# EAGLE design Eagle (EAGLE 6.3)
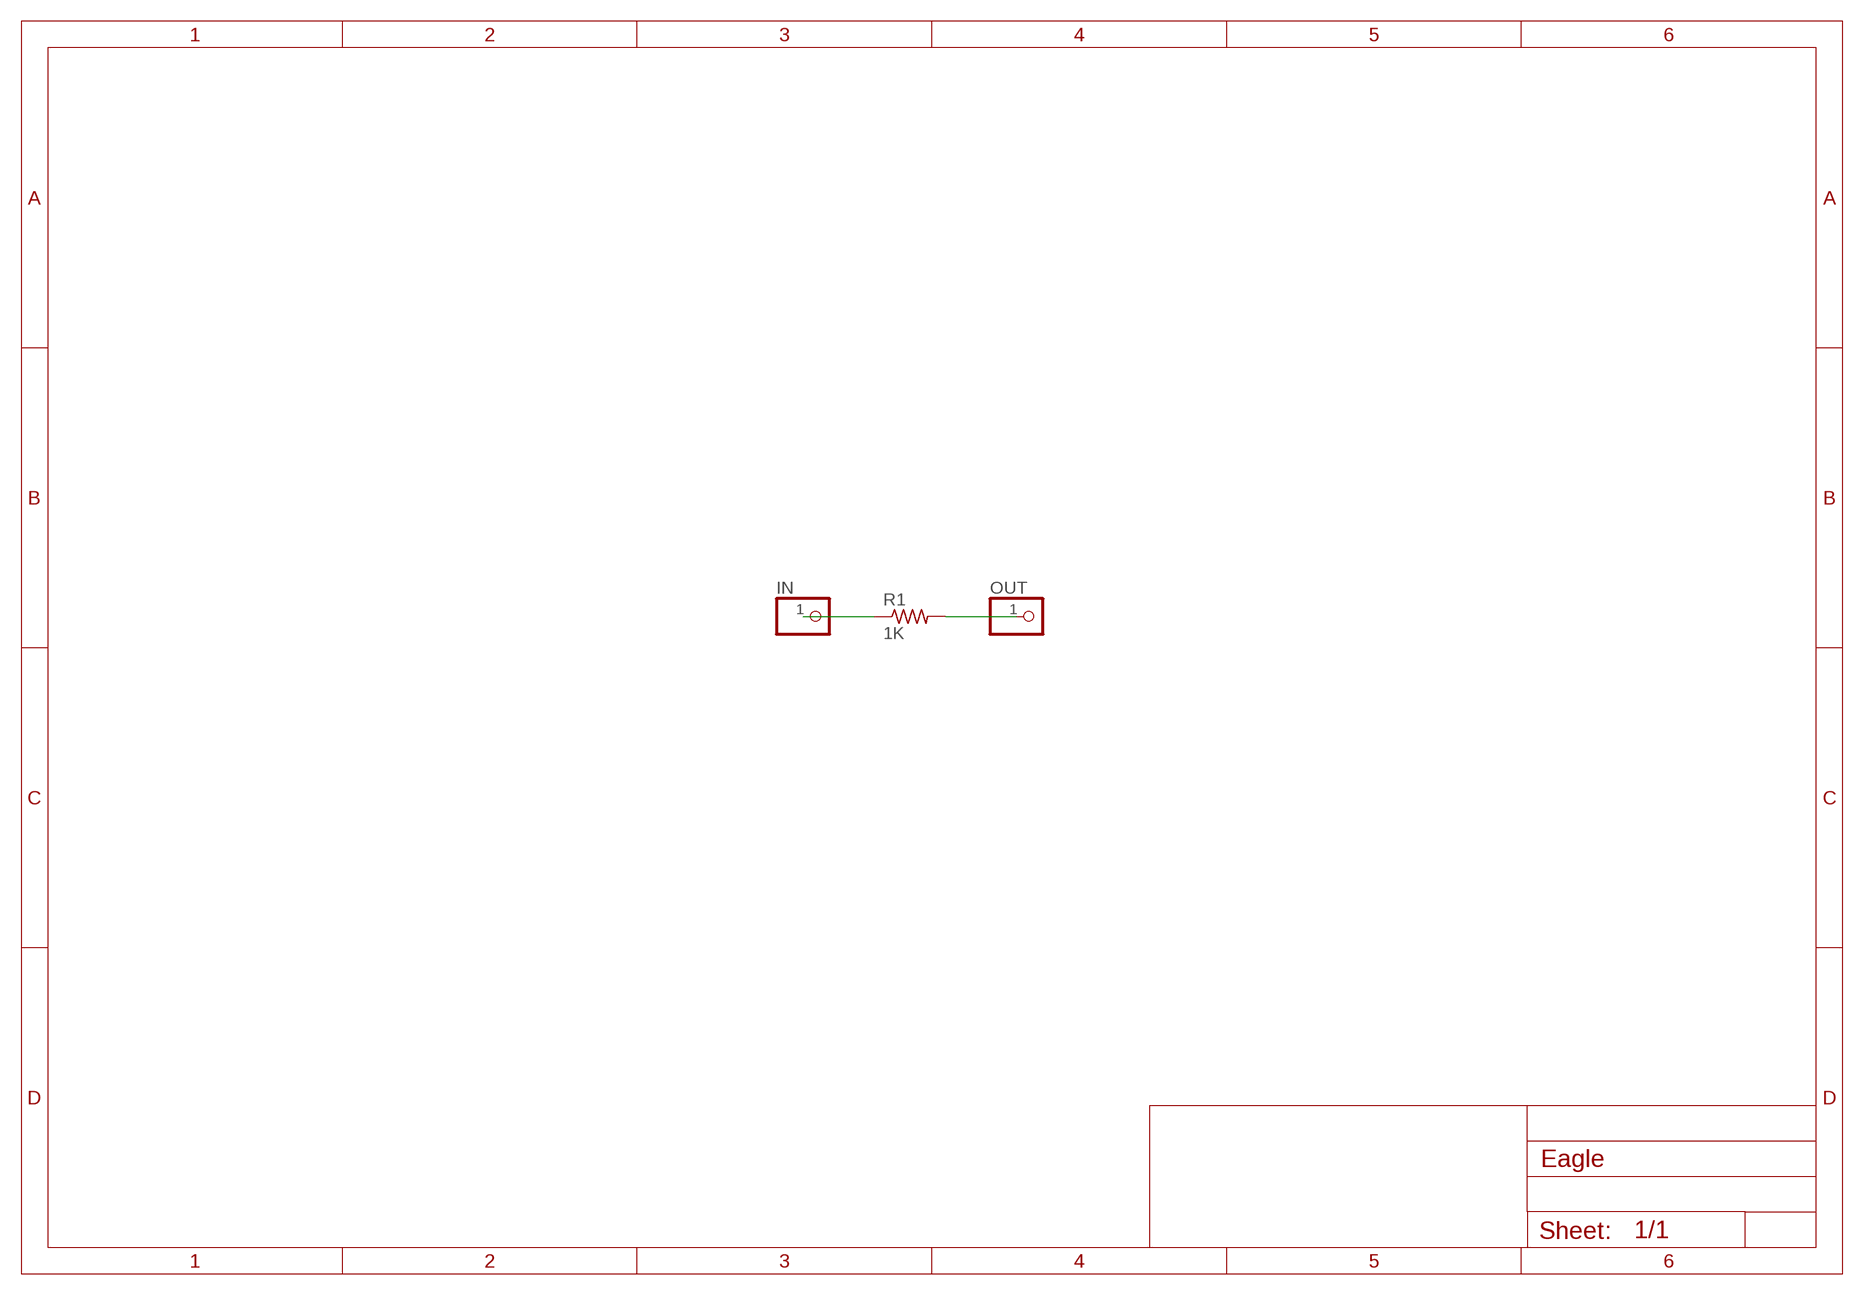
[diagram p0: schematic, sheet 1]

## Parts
IN  PINHD-1X1  [1X01]
OUT  PINHD-1X1  [1X01]
R1  1K  R-US_R0805  [R0805]

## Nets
N$1: IN.1 R1.1
N$2: OUT.1 R1.2

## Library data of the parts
IN OUT = pinhead:PINHD-1X1: PIN HEADER
R1 = rcl:R-US_: RESISTOR, American symbol

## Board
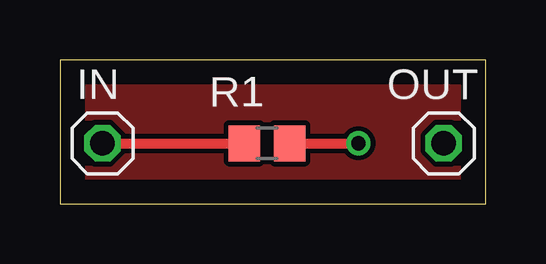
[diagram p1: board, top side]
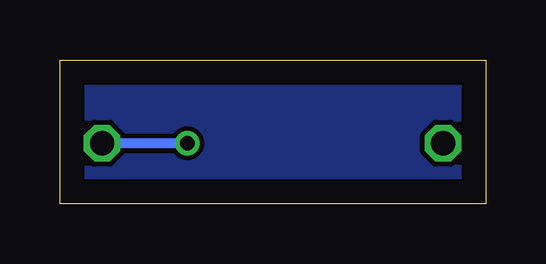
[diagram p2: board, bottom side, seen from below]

Size 17.76 x 6.02 mm. Coordinates in mm from the lower left corner, seen from the top.
Outline: 0,0 17.76,0 17.76,6.02 0,6.02 0,0
Copper layers (1*16): Top 0.035mm / dielectric 1.5mm / Bottom 0.035mm
Design rules "default": minimum track width 10mil, minimum drill 24mil, track to track 8mil, track to pad 8mil, pad to pad 8mil, via to via 8mil, smd to smd 8mil, copper to edge 40mil, drill to drill 8mil, minimum pad ring 10mil, minimum via ring 8mil, stop-mask expansion 4mil, vias tented up to drill 0mil, thermal gap 10mil

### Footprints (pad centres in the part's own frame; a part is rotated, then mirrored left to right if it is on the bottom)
1X01 = drill 1.016 octagon: 1 0,0
R0805 = smd 1.3 x 1.5: 1 -0.95,0; 2 0.95,0

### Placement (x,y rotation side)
IN  1.78,2.54 0 top
OUT  16,2.54 0 top
R1  8.64,2.54 0 top

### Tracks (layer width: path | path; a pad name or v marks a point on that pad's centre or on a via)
GND
  pour Bottom: -0.25,-0.25 -0.25,6.35 18.03,6.35 18.03,-0.25
  pour Top: -0.51,6.6 18.29,6.6 18.29,-0.51 -0.51,-0.51
N$1
  Top 0.406: IN.1 R1.1
N$2  (via drill 0.6)
  Top 0.406: R1.2 v12.45,2.54
  Bottom 0.406: v12.45,2.54 OUT.1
